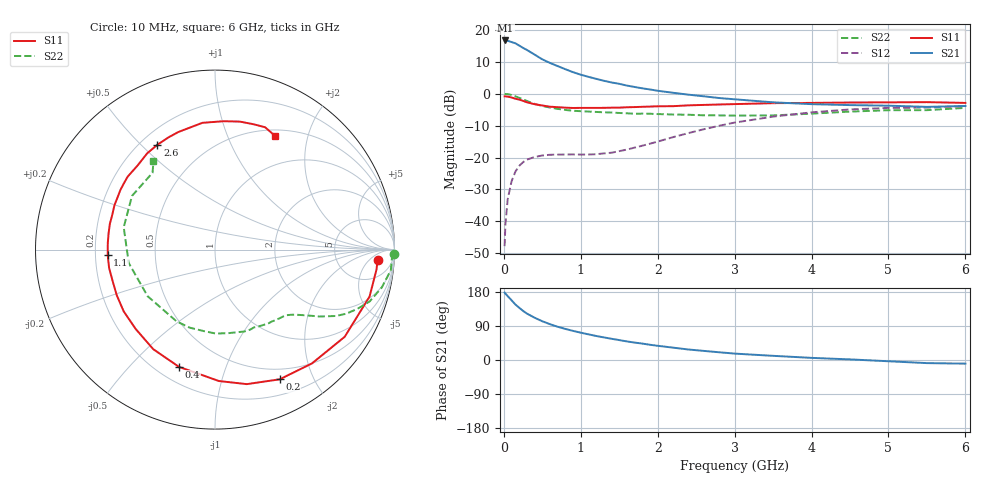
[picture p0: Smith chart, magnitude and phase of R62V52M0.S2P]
! SIEMENS Small Signal Semiconductors
! BFR193
! Si NPN RF Bipolar Junction Transistor in SOT23
! VCE = 2.5 V  IC = 2 mA
! Common Emitter S-Parameters:  May  1996
# GHz  S  MA  R  50
!  f  S11  S21  S12  S22
! GHz  MAG  ANG  MAG  ANG  MAG  ANG  MAG  ANG
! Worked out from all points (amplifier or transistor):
!   36 points, 10 MHz to 6 GHz, reference 50 ohm
!   highest |S21| = 16.7 dB at 20 MHz (marker M1)
!   |S21| within 3 dB of that: start of sweep to 301.5 MHz
!   unconditionally stable (mu >= 1): 1.146 GHz to 2.037 GHz
!   at 250 MHz: K = 0.23, MSG = 17.9 dB, |S12| = -21.4 dB
!   at 1.4 GHz: K = 1.11, MAG = 8.9 dB, |S12| = -18.5 dB
!   at 6 GHz: K = 1.00, MSG = 0.0 dB, |S12| = -3.9 dB
!   S11 on the Smith chart (normalised r, x): 10 MHz: 15, -9; 200 MHz: 0.37, -1.55; 400 MHz: 0.29, -0.70; 1.1 GHz: 0.25, -0.02; 2.6 GHz: 0.27, +0.56; 6 GHz: 0.57, +1.50
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0.01  0.9079 -3.5  6.666 178.0  0.0041 87.8  0.9968 -1.3
0.02  0.9067 -7.0  6.803 175.3  0.0089 88.1  0.9869 -2.7
0.05  0.9 -16.9  6.723 168.6  0.0222 79.7  0.9862 -6.7
0.1  0.8708 -33.9  6.425 157.7  0.0423 71.6  0.9529 -12.8
0.15  0.833 -49.6  6.141 146.5  0.0601 63.4  0.9091 -18.5
0.2  0.8076 -63.5  5.658 137.9  0.074 56.9  0.8594 -22.6
0.25  0.7702 -76.7  5.201 129.6  0.0847 50.8  0.8129 -26.1
0.3  0.7326 -88.3  4.828 122.5  0.0928 46.6  0.7678 -28.8
0.4  0.6833 -107.1  4.086 111.6  0.102 39.9  0.6919 -32.6
0.5  0.6528 -121.8  3.443 102.2  0.1077 35.5  0.6412 -35.0
0.6  0.6251 -135.0  3.025 94.5  0.1105 33.1  0.6063 -37.0
0.7  0.6143 -145.8  2.699 87.7  0.1112 32.1  0.5774 -38.9
0.9  0.5968 -162.7  2.168 76.8  0.1118 33.4  0.5401 -42.6
1.1  0.5986 -177.1  1.833 67.7  0.1116 37.0  0.5244 -47.0
1.3  0.5998 171.2  1.592 59.6  0.1161 43.1  0.5105 -51.8
1.6  0.6122 156.3  1.338 49.0  0.1332 53.3  0.4926 -60.3
2.2  0.637 132.5  1.032 32.6  0.2086 62.8  0.4715 -80.9
2.6  0.6664 118.8  0.909 24.0  0.2776 60.9  0.4582 -98.1
3.5  0.7097 95.7  0.732 11.0  0.4371 45.4  0.4564 -145.3
4.5  0.7265 79.0  0.662 1.6  0.5665 24.6  0.5236 166.2
5.5  0.7365 67.7  0.621 -8.2  0.6046 5.6  0.5518 129.1
6  0.7167 62.3  0.641 -9.6  0.6383 0.3  0.5991 124.9
